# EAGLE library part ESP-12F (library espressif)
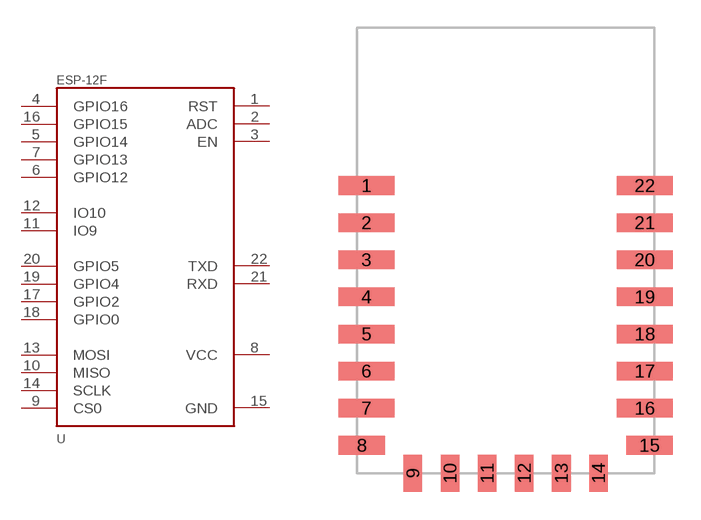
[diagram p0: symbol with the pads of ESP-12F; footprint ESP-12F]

Designator prefix -

## ESP-12F  [ESP-12F]
1  RST
2  ADC
3  EN
4  GPIO16
5  GPIO14
6  GPIO12
7  GPIO13
8  VCC
9  CS0
10  MISO
11  IO9
12  IO10
13  MOSI
14  SCLK
15  GND
16  GPIO15
17  GPIO2
18  GPIO0
19  GPIO4
20  GPIO5
21  RXD
22  TXD

## Footprint ESP-12F (pad centres in mm)
smd 3 x 1: 1 -7.5,-8.5; 2 -7.5,-10.5; 3 -7.5,-12.5; 4 -7.5,-14.5; 5 -7.5,-16.5; 6 -7.5,-18.5; 7 -7.5,-20.5; 16 7.5,-20.5; 17 7.5,-18.5; 18 7.5,-16.5; 19 7.5,-14.5; 20 7.5,-12.5; 21 7.5,-10.5; 22 7.5,-8.5
smd 2.5 x 1: 8 -7.75,-22.5; 15 7.75,-22.5
smd 1 x 2: 9 -5,-24; 10 -3,-24; 11 -1,-24; 12 1,-24; 13 3,-24; 14 5,-24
